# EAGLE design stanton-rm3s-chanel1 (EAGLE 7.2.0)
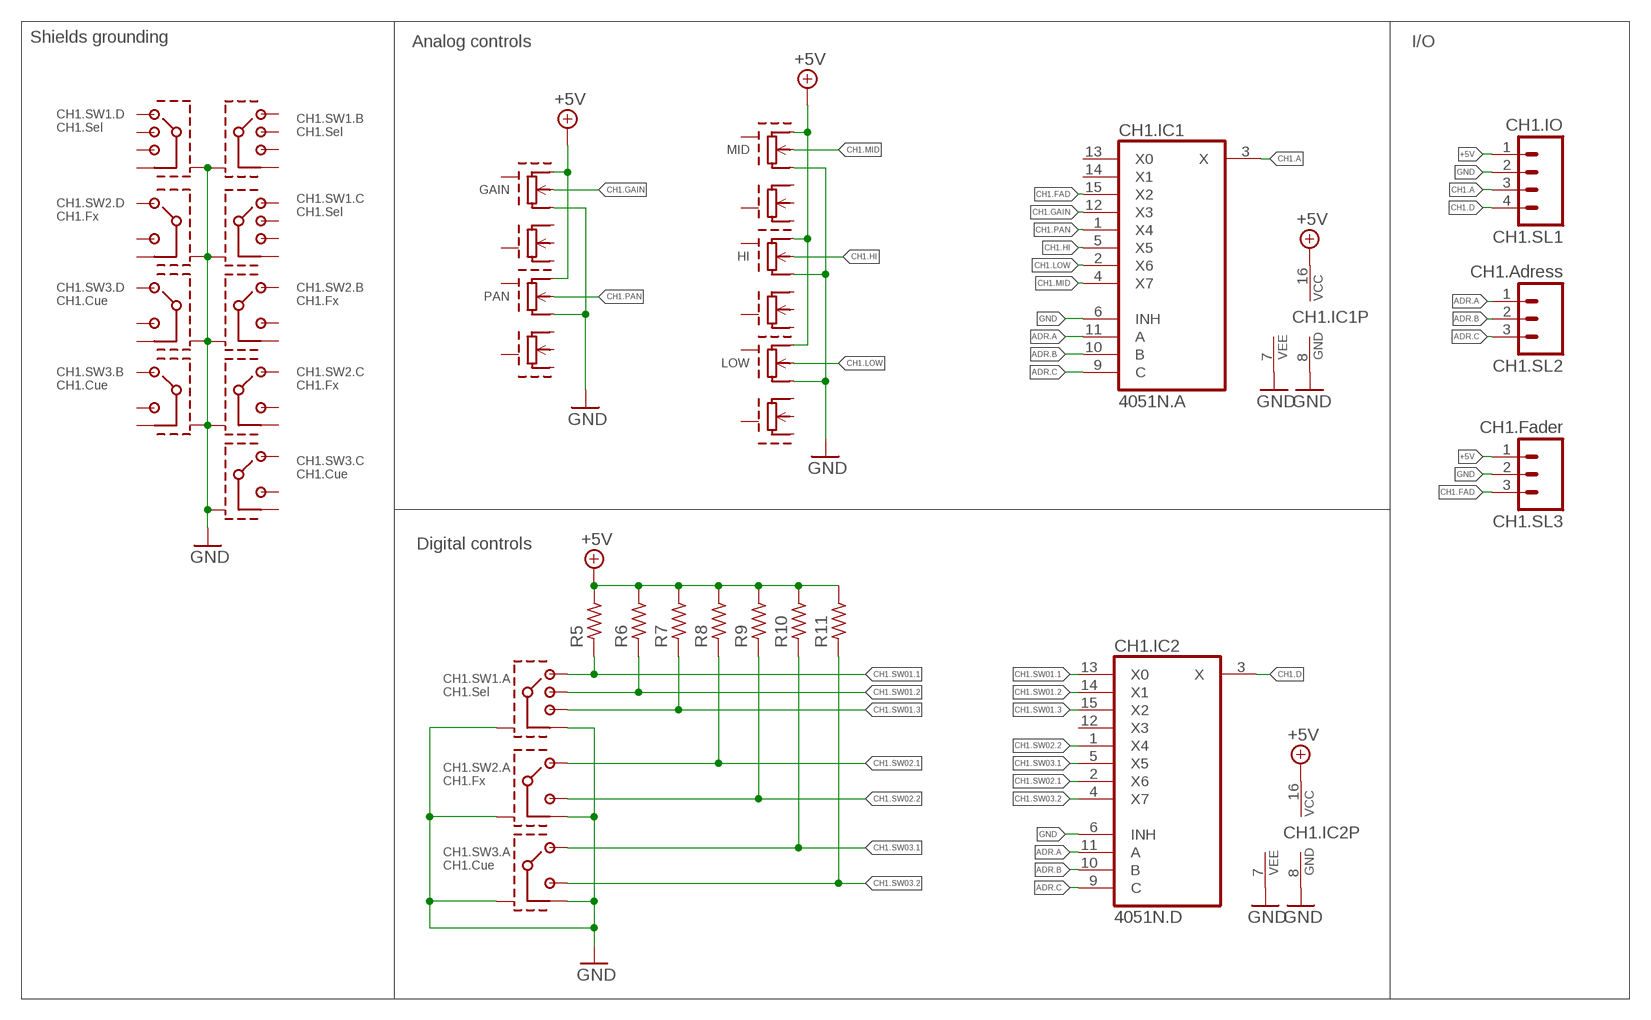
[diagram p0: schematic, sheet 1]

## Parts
CH1.IC1  4051N.A  4051N  [DIL16]
CH1.IC2  4051N.D  4051N  [DIL16]
CH1.SL1  CH1.IO  M04  [04P]
CH1.SL2  CH1.Adress  M03  [03P]
CH1.SL3  CH1.Fader  M03  [03P]
CH1.SW1.  CH1.Sel  RM3S-2P-SWITCH  [RM3S-2P-SWITCH]
CH1.SW2.  CH1.Fx  RM3S-1P-SWITCH  [RM3S-1P-SWITCH]
CH1.SW3.  CH1.Cue  RM3S-1P-SWITCH  [RM3S-1P-SWITCH]
GAIN  RM3S-POTRM3S-POT  [RM3S-POT]
HI  RM3S-POTRM3S-POT  [RM3S-POT]
LOW  RM3S-POTRM3S-POT  [RM3S-POT]
MID  RM3S-POTRM3S-POT  [RM3S-POT]
PAN  RM3S-POTRM3S-POT  [RM3S-POT]
R5  R-EU_0207/10C  [0207/10C]
R6  R-EU_0207/10C  [0207/10C]
R7  R-EU_0207/10C  [0207/10C]
R8  R-EU_0207/10C  [0207/10C]
R9  R-EU_0207/10C  [0207/10C]
R10  R-EU_0207/10C  [0207/10C]
R11  R-EU_0207/10C  [0207/10C]

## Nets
+5V: CH1.IC1.16(VCC) CH1.IC2.16(VCC) CH1.SL1.1 CH1.SL3.1 GAIN.1 HI.1 LOW.1 MID.1 PAN.1 R5.2 R6.2 R7.2 R8.2 R9.2 R10.2 R11.2
ADR.A: CH1.IC1.11(A) CH1.IC2.11(A) CH1.SL2.1
ADR.B: CH1.IC1.10(B) CH1.IC2.10(B) CH1.SL2.2
ADR.C: CH1.IC1.9(C) CH1.IC2.9(C) CH1.SL2.3
CH1.A: CH1.IC1.3(X) CH1.SL1.3
CH1.D: CH1.IC2.3(X) CH1.SL1.4
CH1.FAD: CH1.IC1.15(X2) CH1.SL3.3
CH1.GAIN: CH1.IC1.12(X3) GAIN.6
CH1.HI: CH1.IC1.5(X5) HI.6
CH1.LOW: CH1.IC1.2(X6) LOW.6
CH1.MID: CH1.IC1.4(X7) MID.6
CH1.PAN: CH1.IC1.1(X4) PAN.6
CH1.SW01.1: CH1.IC2.13(X0) CH1.SW1..1.1 R5.1
CH1.SW01.2: CH1.IC2.14(X1) CH1.SW1..1.2 R6.1
CH1.SW01.3: CH1.IC2.15(X2) CH1.SW1..1.3 R7.1
CH1.SW02.1: CH1.IC2.2(X6) CH1.SW2..1.1 R8.1
CH1.SW02.2: CH1.IC2.1(X4) CH1.SW2..1.3 R9.1
CH1.SW03.1: CH1.IC2.5(X5) CH1.SW3..1.1 R10.1
CH1.SW03.2: CH1.IC2.4(X7) CH1.SW3..1.3 R11.1
GND: CH1.IC1.6(INH) CH1.IC1.7(VEE) CH1.IC1.8(GND) CH1.IC2.6(INH) CH1.IC2.7(VEE) CH1.IC2.8(GND) CH1.SL1.2 CH1.SL3.2 CH1.SW1..1.4 CH1.SW1..GND1(A:GND1) CH1.SW1..GND2(B:GND1) CH1.SW1..GND3(C:GND1) CH1.SW1..GND4(D:GND1) CH1.SW2..1.4 CH1.SW2..P$13(A:GND1) CH1.SW2..P$14(B:GND1) CH1.SW2..P$15(C:GND1) CH1.SW2..P$16(D:GND1) CH1.SW3..1.4 CH1.SW3..P$13(A:GND1) CH1.SW3..P$14(B:GND1) CH1.SW3..P$15(C:GND1) CH1.SW3..P$16(D:GND1) GAIN.5 HI.5 LOW.5 MID.5 PAN.5
Unconnected: CH1.IC1.13(X0) CH1.IC1.14(X1) CH1.IC2.12(X3) CH1.SW1..2.1 CH1.SW1..2.2 CH1.SW1..2.3 CH1.SW1..2.4 CH1.SW1..3.1 CH1.SW1..3.2 CH1.SW1..3.3 CH1.SW1..3.4 CH1.SW1..4.1 CH1.SW1..4.2 CH1.SW1..4.3 CH1.SW1..4.4 CH1.SW2..2.1 CH1.SW2..2.3 CH1.SW2..2.4 CH1.SW2..3.1 CH1.SW2..3.3 CH1.SW2..3.4 CH1.SW2..4.1 CH1.SW2..4.3 CH1.SW2..4.4 CH1.SW3..2.1 CH1.SW3..2.3 CH1.SW3..2.4 CH1.SW3..3.1 CH1.SW3..3.3 CH1.SW3..3.4 CH1.SW3..4.1 CH1.SW3..4.3 CH1.SW3..4.4 GAIN.2 GAIN.3 GAIN.4 GAIN.GND1 GAIN.GND2 HI.2 HI.3 HI.4 HI.GND1 HI.GND2 LOW.2 LOW.3 LOW.4 LOW.GND1 LOW.GND2 MID.2 MID.3 MID.4 MID.GND1 MID.GND2 PAN.2 PAN.3 PAN.4 PAN.GND1 PAN.GND2

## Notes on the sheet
- Shields grounding | Analog controls | I/O
- Digital controls

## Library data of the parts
CH1.IC1 CH1.IC2 = 40xx:4051: 8-channel ANALOG MULTIPLEXER
CH1.SL1 = con-amp-quick:M04: AMP QUICK CONNECTOR
CH1.SL2 CH1.SL3 = con-amp-quick:M03: AMP QUICK CONNECTOR
CH1.SW1. = stanton-rm3s:RM3S-2P-SWITCH
CH1.SW2. CH1.SW3. = stanton-rm3s:RM3S-1P-SWITCH
GAIN HI LOW MID PAN = stanton-rm3s:RM3S-POT
R5-R11 = rcl:R-EU_: RESISTOR, European symbol

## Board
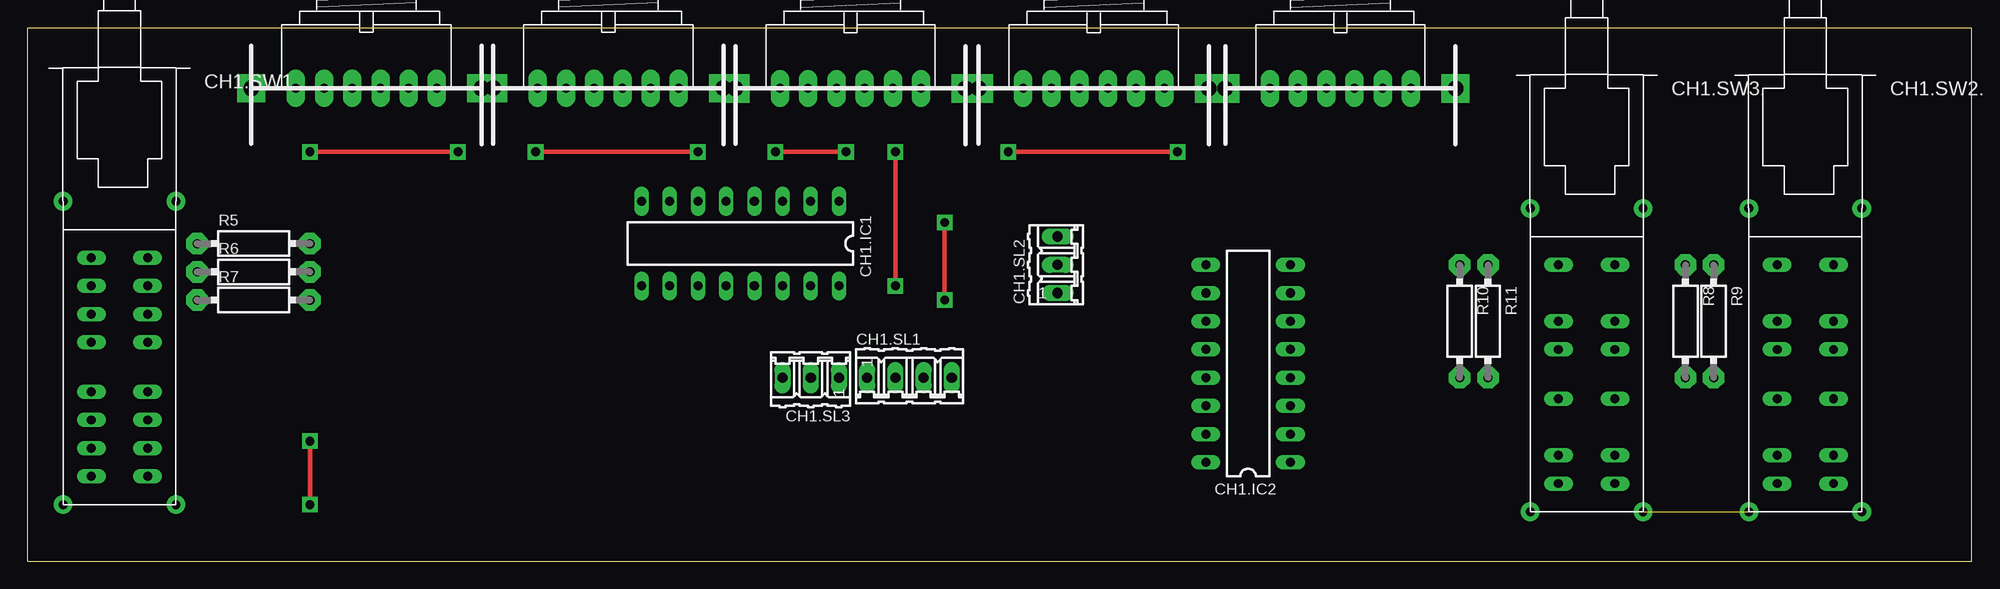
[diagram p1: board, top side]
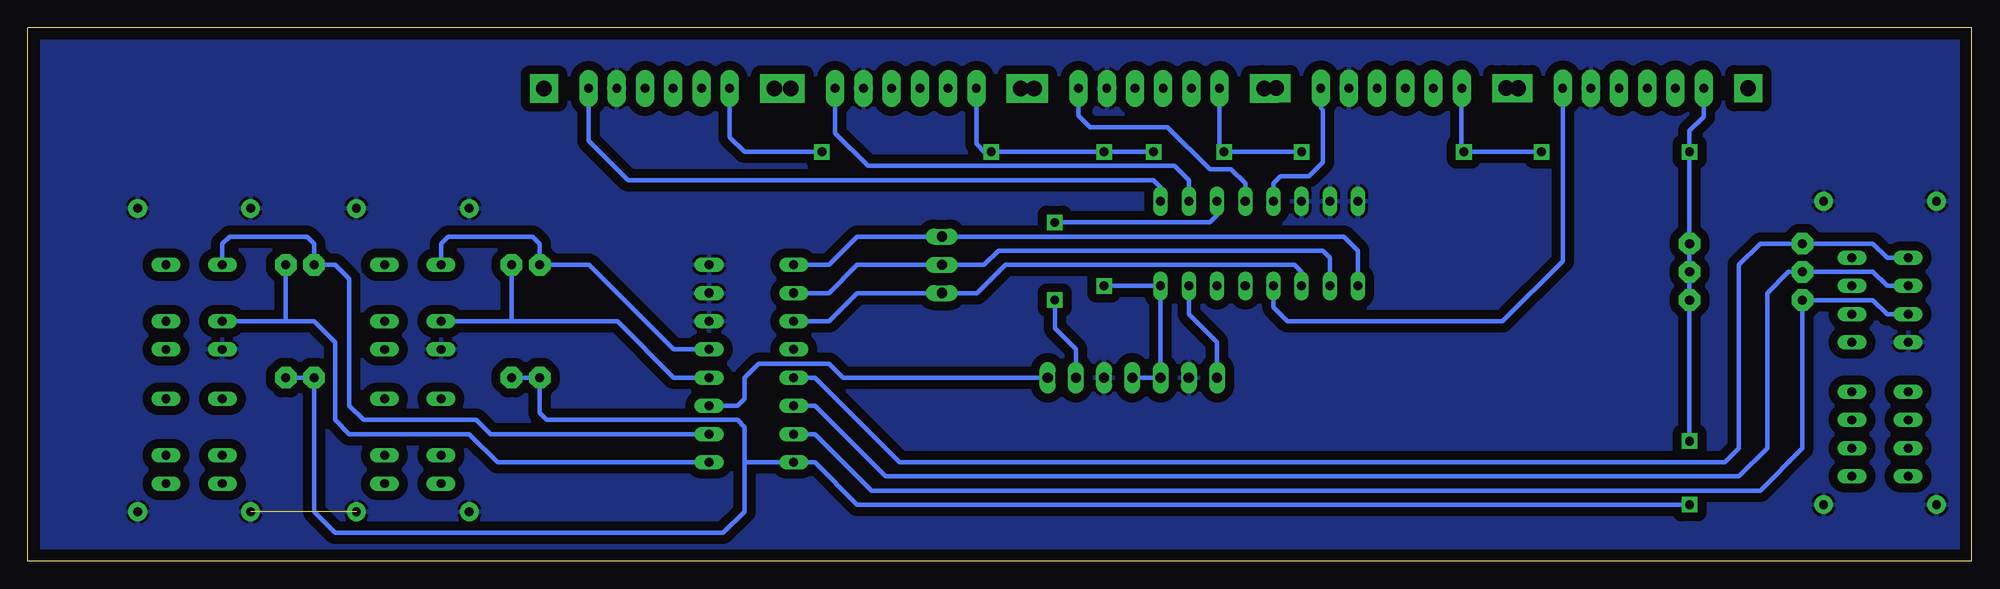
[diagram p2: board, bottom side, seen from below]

Size 175 x 48 mm. Coordinates in mm from the lower left corner, seen from the top.
Outline: 0,0 0,48 175,48 175,0 0,0
Copper layers (1*16): Top 0.035mm / dielectric 1.5mm / Bottom 0.035mm
Design rules "default": minimum track width 10mil, minimum drill 24mil, track to track 8mil, track to pad 8mil, pad to pad 8mil, via to via 8mil, smd to smd 8mil, copper to edge 40mil, drill to drill 8mil, minimum pad ring 10mil, minimum via ring 8mil, stop-mask expansion 4mil, vias tented up to drill 0mil, thermal gap 10mil

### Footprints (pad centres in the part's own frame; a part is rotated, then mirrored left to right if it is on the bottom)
DIL16 = drill 0.813 long: 1 -8.89,-3.81; 2 -6.35,-3.81; 3 -3.81,-3.81; 4 -1.27,-3.81; 5 1.27,-3.81; 6 3.81,-3.81; 7 6.35,-3.81; 8 8.89,-3.81; 9 8.89,3.81; 10 6.35,3.81; 11 3.81,3.81; 12 1.27,3.81; 13 -1.27,3.81; 14 -3.81,3.81; 15 -6.35,3.81; 16 -8.89,3.81
04P = drill 0.914 long: 1 -3.81,0; 2 -1.27,0; 3 1.27,0; 4 3.81,0
03P = drill 0.914 long: 1 -2.54,0; 2 0,0; 3 2.54,0
RM3S-2P-SWITCH = drill 0.8 long: 1.1 -2.54,0; 1.2 -2.54,-2.54; 1.3 -2.54,-5.08; 1.4 -2.54,-7.62; 2.1 2.54,0; 2.2 2.54,-2.54; 2.3 2.54,-5.08; 2.4 2.54,-7.62; 3.1 -2.54,-12.065; 3.2 -2.54,-14.605; 3.3 -2.54,-17.145; 3.4 -2.54,-19.685; 4.1 2.54,-12.065; 4.2 2.54,-14.605; 4.3 2.54,-17.145; 4.4 2.54,-19.685 | drill 0.8 pad 1.676: GND1 -5.08,5.08; GND2 5.08,5.08; GND3 -5.08,-22.225; GND4 5.08,-22.225
RM3S-1P-SWITCH = drill 0.8 long: 1.1 -2.54,0; 1.3 -2.54,-5.08; 1.4 -2.54,-7.62; 2.1 2.54,0; 2.3 2.54,-5.08; 2.4 2.54,-7.62; 3.1 -2.54,-12.065; 3.3 -2.54,-17.145; 3.4 -2.54,-19.685; 4.1 2.54,-12.065; 4.3 2.54,-17.145; 4.4 2.54,-19.685 | drill 0.8 pad 1.676: P$13 -5.08,-22.225; P$14 5.08,-22.225; P$15 -5.08,5.08; P$16 5.08,5.08
RM3S-POT = drill 0.8 pad 1.676 long: 1 -6.35,0; 2 -3.81,0; 3 -1.27,0; 4 1.27,0; 5 3.81,0; 6 6.35,0 | drill 1.4 pad 2.54 square: GND1 -10.36,0; GND2 10.36,0
0207/10C = drill 0.813 pad 1.93 octagon: 1 -5.08,0; 2 5.08,0

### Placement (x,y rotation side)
CH1.IC1  64.14,28.57 180 top
CH1.IC2  109.86,17.78 90 top
CH1.SL1  79.38,16.51 0 top
CH1.SL2  92.71,26.67 90 top
CH1.SL3  70.48,16.51 180 top
CH1.SW1.  8.26,27.31 0 top
CH1.SW2.  160.02,26.67 0 top
CH1.SW3.  140.34,26.67 0 top
GAIN  30.48,42.56 0 top
HI  52.26,42.56 0 top
LOW  95.96,42.54 0 top
MID  74.06,42.54 0 top
PAN  118.16,42.54 0 top
R5  20.32,28.57 0 top
R6  20.32,26.03 0 top
R7  20.32,23.5 0 top
R8  149.22,21.59 270 top
R9  151.76,21.59 270 top
R10  128.91,21.59 270 top
R11  131.44,21.59 270 top

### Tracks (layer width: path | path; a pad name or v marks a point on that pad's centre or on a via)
+5V  (via drill 0.8 pad 1.4)
  Top 0.406: v103.5,36.83 v88.27,36.83 | v73.66,36.83 v67.31,36.83 | v60.33,36.83 v45.72,36.83 | v78.11,36.83 v78.11,24.77 | v25.4,5.08 v25.4,10.8 | v38.73,36.83 v25.4,36.83
  Bottom 0.4: 110.49,8.89 CH1.IC2.16 104.14,8.89 100.33,5.08 v25.4,5.08 | R11.2 R10.2 128.91,13.33 128.27,12.7 111.12,12.7 110.49,12.06 110.49,8.89 | 110.49,8.89 110.49,4.44 112.39,2.54 147.32,2.54 149.22,4.44 R8.2 R9.2 | 111.81,38.15 110.49,36.83 v103.5,36.83 | v60.33,36.83 v67.31,36.83 67.72,37.24 | v73.66,36.83 v78.11,36.83 v88.27,36.83 88.9,36.83 89.61,37.54 | v78.11,24.77 CH1.IC1.16 CH1.SL3.1 CH1.SL1.1 | 24.13,40 25.4,38.74 v25.4,36.83 R5.2 R6.2 R7.2 v25.4,10.8 | 45.92,37.03 v45.72,36.83 v38.73,36.83
  Bottom 0.406: 24.13,40 GAIN.1 | 45.92,37.03 45.92,42.54 HI.1 | MID.1 67.71,37.25 67.72,37.24 | LOW.1 89.61,38.18 89.61,37.54 | 111.81,38.15 PAN.1
ADR.A
  Bottom 0.4: CH1.IC1.11 60.33,26.03 60.96,26.67 87,26.67 89.53,24.13 CH1.SL2.1 100.33,24.13 102.87,21.59 CH1.IC2.11
ADR.B
  Bottom 0.4: CH1.IC1.10 57.78,27.31 58.42,27.94 87.63,27.94 88.9,26.67 CH1.SL2.2 100.33,26.67 102.87,24.13 CH1.IC2.10
ADR.C
  Bottom 0.4: CH1.IC1.9 55.24,27.94 56.52,29.21 CH1.SL2.3 100.33,29.21 102.87,26.67 CH1.IC2.9
CH1.A  (via drill 0.8 pad 1.4)
  Top 0.406: v82.55,30.48 v82.55,23.5
  Bottom 0.4: CH1.IC1.3 67.94,31.12 68.58,30.48 v82.55,30.48 | v82.55,23.5 82.55,20.95 80.64,19.05 CH1.SL1.3
CH1.D
  Bottom 0.4: CH1.SL1.4 101.6,16.51 102.87,17.78 109.22,17.78 110.49,16.51 110.49,14.61 111.12,13.97 CH1.IC2.3
CH1.FAD
  Bottom 0.4: CH1.SL3.3 67.94,19.69 70.48,22.22 CH1.IC1.15
CH1.GAIN
  Bottom 0.4: 61.59,21.59 62.87,22.86 CH1.IC1.12
  Bottom 0.406: GAIN.6 36.83,27 42.24,21.59 61.59,21.59
CH1.HI
  Bottom 0.406: HI.6 58.61,40.78 58.42,40.59 58.42,35.89 59.69,34.62 62.23,34.62 62.87,33.99 CH1.IC1.5
CH1.LOW
  Bottom 0.4: CH1.IC1.2 70.48,34.29 71.75,35.56 90.81,35.56
  Bottom 0.406: 90.81,35.56 99.36,35.56 102.31,38.51 LOW.6
CH1.MID
  Bottom 0.406: CH1.IC1.4 65.41,33.99 66.67,35.25 68.58,35.25 72.39,39.06 79.38,39.06 80.41,40.1 MID.6
CH1.PAN
  Bottom 0.4: CH1.IC1.1 73.03,33.66 73.66,34.29 112.39,34.29
  Bottom 0.406: 112.39,34.29 120.95,34.29 124.51,37.85 PAN.6
CH1.SW01.1
  Bottom 0.4: CH1.SW1..1.1 7.62,27.31 8.89,28.57 R5.1 19.05,28.57 20.95,26.67 20.95,10.16 22.23,8.89 96.52,8.89 104.14,16.51 CH1.IC2.13
CH1.SW01.2
  Bottom 0.4: CH1.SW1..1.2 7.62,24.77 8.89,26.03 R6.1 16.51,26.03 18.41,24.13 18.41,10.16 20.95,7.62 97.79,7.62 104.14,13.97 CH1.IC2.14
CH1.SW01.3
  Bottom 0.4: CH1.SW1..1.3 7.62,22.22 8.89,23.5 R7.1 15.24,10.16 19.05,6.35 99.06,6.35 104.14,11.43 CH1.IC2.15
CH1.SW02.1
  Bottom 0.4: CH1.SW2..1.1 157.48,28.57 156.84,29.21 149.86,29.21 149.22,28.57 R8.1 147.32,26.67 146.05,25.4 146.05,13.97 144.78,12.7 134.62,12.7 133.35,11.43 CH1.IC2.2
CH1.SW02.2
  Bottom 0.4: CH1.SW2..1.3 151.76,21.59 | R9.1 151.76,21.59 | 151.76,21.59 149.22,21.59 147.32,19.69 147.32,12.7 146.05,11.43 135.25,11.43 132.72,8.89 CH1.IC2.1
CH1.SW03.1
  Bottom 0.4: CH1.SW3..1.1 137.79,28.57 137.16,29.21 129.54,29.21 128.91,28.57 R10.1 124.46,26.67 116.84,19.05 CH1.IC2.5
CH1.SW03.2
  Bottom 0.4: CH1.SW3..1.3 131.44,21.59 | 131.44,21.59 R11.1 | CH1.IC2.4 116.84,16.51 121.92,21.59 131.44,21.59
GND  (1 unrouted)
  pour Bottom (isolate 0.813): 0.64,47.53 0.64,0.64 173.99,0.64 173.99,47.53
